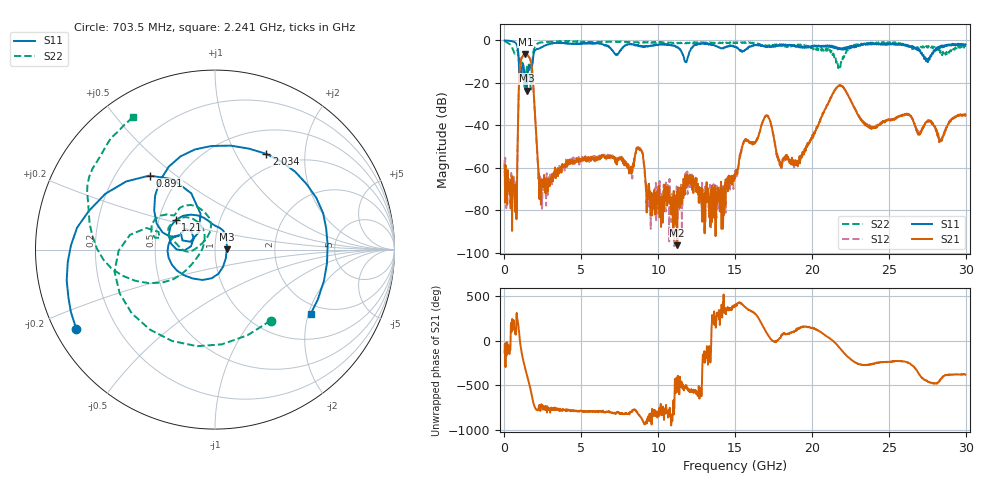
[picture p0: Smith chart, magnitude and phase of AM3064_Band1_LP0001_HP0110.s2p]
# Hz S DB R 50.0
!freq dBS11 angS11 dBS21 angS21 dBS12 angS12 dBS22 angS22
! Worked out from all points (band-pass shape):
!   1600 points, 10 MHz to 29.98 GHz, reference 50 ohm
!   highest |S21| = -6.34 dB at 1.36 GHz (marker M1); lowest = -96.6 dB at 11.24 GHz (marker M2)
!   |S21| within 3 dB of the highest: 1.077 GHz to 1.691 GHz (613.9 MHz wide, 44.4 % of centre)
!   lowest |S11| = -23.6 dB at 1.435 GHz (marker M3), VSWR 1.14, Z = 57.1 + j0.214 ohm
!   |S11| at or under -10 dB: 931.4 MHz to 1.831 GHz (899.7 MHz wide, 65.1 % of centre); 11.75 GHz to 11.85 GHz (94.01 MHz wide, 0.797 % of centre); 27.52075 GHz to 27.54983 GHz (29.08 MHz wide, 0.106 % of centre)
!   |S22| runs from -23.1 to -0.2 dB; largest |S21 - S12| = 0.0044
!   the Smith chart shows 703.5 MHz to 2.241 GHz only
!   S11 on the Smith chart (normalised r, x): 703.5 MHz: 0.06, -0.26; 891 MHz: 0.34, +0.41; 1.21 GHz: 0.61, +0.22; 2.034 GHz: 0.80, +1.34; 2.241 GHz: 1.69, -2.07
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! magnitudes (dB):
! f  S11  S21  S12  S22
! 10 MHz  0.0  -58.5  -56.5  -0.2
! 703.5 MHz  -1.0  -68.6  -70.8  -6.0
! 891 MHz  -5.2  -35.7  -35.7  -6.4
! 1.21 GHz  -11.2  -7.2  -7.2  -11.9
! 1.36 GHz  -18.1  -6.3  -6.3  -18.1
! 1.435 GHz  -23.6  -6.5  -6.4  -13.8
! 1.753 GHz  -13.3  -11.3  -11.3  -17.1
! 2.034 GHz  -4.4  -41.0  -40.9  -2.2
! 2.241 GHz  -3.8  -62.8  -65.6  -1.2
! 5.015 GHz  -1.5  -56.1  -56.8  -0.7
! 8.745 GHz  -2.7  -51.3  -50.4  -1.1
! 9.363 GHz  -2.7  -73.7  -74.7  -1.0
! 10 GHz  -2.0  -70.3  -72.7  -0.9
! 11.24 GHz  -3.4  -96.6  -75.1  -1.3
! 15 GHz  -3.1  -62.7  -61.4  -1.3
! 17.01 GHz  -3.2  -35.5  -35.4  -2.5
! 17.95 GHz  -2.3  -57.6  -57.7  -2.0
! 19.99 GHz  -3.1  -46.2  -45.8  -3.4
! 21.81 GHz  -4.1  -21.2  -21.3  -12.6
! 25 GHz  -1.4  -37.5  -37.5  -1.1
! 28.37 GHz  -3.2  -47.2  -47.2  -5.6
! 29.98 GHz  -1.9  -35.1  -35.0  -3.1
